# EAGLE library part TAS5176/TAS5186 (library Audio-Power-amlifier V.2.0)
The TAS5176/TAS5186 is a high-performance, six-channel, digital-amplifier power stage with an improved protection system.
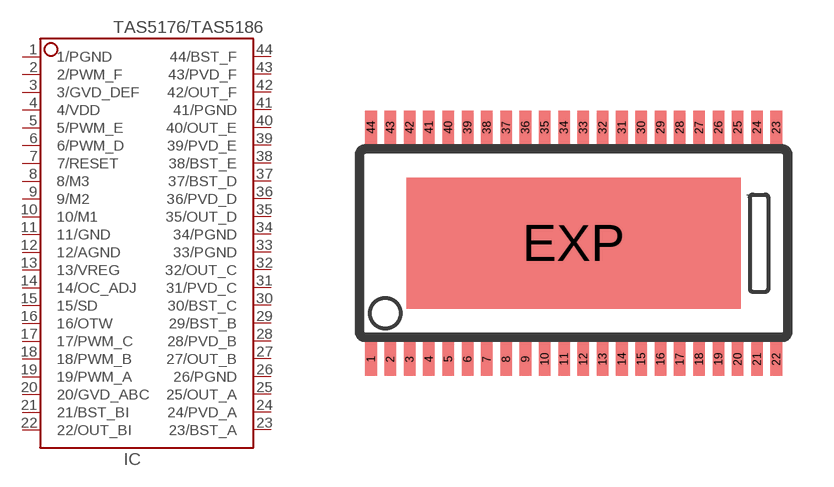
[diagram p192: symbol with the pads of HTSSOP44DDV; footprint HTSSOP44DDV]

Designator prefix IC

## TAS5176/TAS5186  [HTSSOP44DDV]
1  1/PGND  pwr
2  2/PWM_F  in
3  3/GVD_DEF  pwr
4  4/VDD  pwr
5  5/PWM_E  in
6  6/PWM_D  in
7  7/RESET  in
8  8/M3  in
9  9/M2  in
10  10/M1  in
11  11/GND  pwr
12  12/AGND  pwr
13  13/VREG  out
14  14/OC_ADJ  out
15  15/SD  out
16  16/OTW  out
17  17/PWM_C  in
18  18/PWM_B  in
19  19/PWM_A  in
20  20/GVD_ABC  pwr
21  21/BST_BI  pwr
22  22/OUT_BI  out
23  23/BST_A  pwr
24  24/PVD_A  pwr
25  25/OUT_A  out
26  26/PGND  pwr
27  27/OUT_B  out
28  28/PVD_B  pwr
29  29/BST_B  pwr
30  30/BST_C  pwr
31  31/PVD_C  pwr
32  32/OUT_C  out
33  33/PGND  pwr
34  34/PGND  pwr
35  35/OUT_D  out
36  36/PVD_D  pwr
37  37/BST_D  pwr
38  38/BST_E  pwr
39  39/PVD_E  pwr
40  40/OUT_E  out
41  41/PGND  pwr
42  42/OUT_F  out
43  43/PVD_F  pwr
44  44/BST_F  pwr

## Footprint HTSSOP44DDV (pad centres in mm)
PowerPAD(TM) PLASTIC SMALL-OUTLINE PACKAGE DDV (R-PDSO-G**) Source: http://focus.ti.com/lit/ml/mpds041b/mpds041b.pdf / slma002.pdf
smd 0.38 x 1.1: 1 -6.668,-3.81; 2 -6.032,-3.81; 3 -5.397,-3.81; 4 -4.763,-3.81; 5 -4.128,-3.81; 6 -3.493,-3.81; 7 -2.857,-3.81; 8 -2.223,-3.81; 9 -1.587,-3.81; 10 -0.953,-3.81; 11 -0.318,-3.81; 12 0.318,-3.81; 13 0.953,-3.81; 14 1.587,-3.81; 15 2.223,-3.81; 16 2.857,-3.81; 17 3.493,-3.81; 18 4.128,-3.81; 19 4.763,-3.81; 20 5.397,-3.81; 21 6.032,-3.81; 22 6.668,-3.81; 23 6.668,3.81; 24 6.032,3.81; 25 5.397,3.81; 26 4.763,3.81; 27 4.128,3.81; 28 3.493,3.81; 29 2.857,3.81; 30 2.223,3.81; 31 1.587,3.81; 32 0.953,3.81; 33 0.318,3.81; 34 -0.318,3.81; 35 -0.953,3.81; 36 -1.587,3.81; 37 -2.223,3.81; 38 -2.857,3.81; 39 -3.493,3.81; 40 -4.128,3.81; 41 -4.763,3.81; 42 -5.397,3.81; 43 -6.032,3.81; 44 -6.668,3.81
smd 11 x 4.3: EXP 0,0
